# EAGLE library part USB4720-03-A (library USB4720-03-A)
USB Connectors USB2.0 TypeC Recpt., 3u Gold, 16P Horz Mid Mount SMT, 1.13mm O-set, IP67 Source: Datasheet
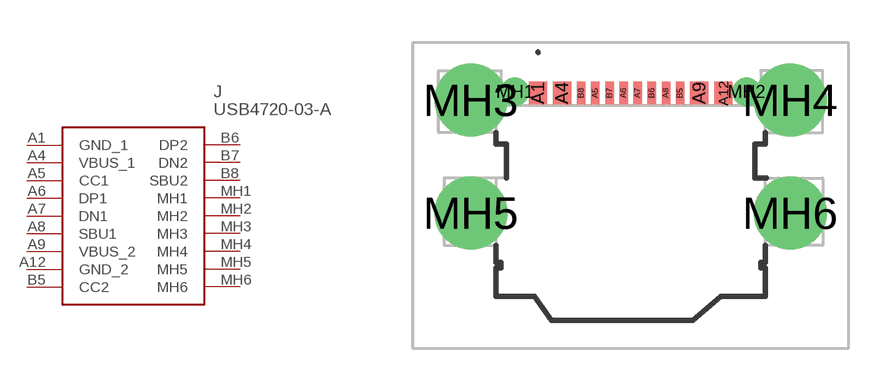
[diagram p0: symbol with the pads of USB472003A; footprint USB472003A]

Designator prefix J

## USB4720-03-A (Description: USB Connectors USB2.0 TypeC Recpt., 3u Gold, 16P Horz Mid Mount SMT, 1.13mm O-set, IP67; Height: 3.9mm; Manufacturer_Name: GCT (GLOBAL CONNECTOR TECHNOLOGY); Manufacturer_Part_Number: USB4720-03-A; Mouser_Part_Number: 640-USB472003A; Mouser_Price-Stock: https://www.mouser.co.uk/ProductDetail/GCT/USB4720-03-A?qs=Z%252BL2brAPG1IK%252BbxHmYg8zQ%3D%3D)  [USB472003A]
A1  GND_1
A4  VBUS_1
A5  CC1
A6  DP1
A7  DN1
A8  SBU1
A9  VBUS_2
A12  GND_2
B5  CC2
B6  DP2
B7  DN2
B8  SBU2
MH1  MH1
MH2  MH2
MH3  MH3
MH4  MH4
MH5  MH5
MH6  MH6

## Footprint USB472003A (pad centres in mm)
USB4720-03-A-1
smd 0.65 x 0.8: A1 -3.28,4; A4 -2.43,4; A9 2.43,4; A12 3.28,4
smd 0.3 x 0.8: A5 -1.25,4; A6 -0.25,4; A7 0.25,4; A8 1.25,4; B5 1.75,4; B6 0.75,4; B7 -0.75,4; B8 -1.75,4
drill 0.5 pad 0.8: MH1 -4.1,4.05; MH2 4.1,4.05
drill 1.72 pad 2.1: MH3 -5.65,3.75; MH4 5.65,3.75; MH5 -5.65,-0.25; MH6 5.65,-0.25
